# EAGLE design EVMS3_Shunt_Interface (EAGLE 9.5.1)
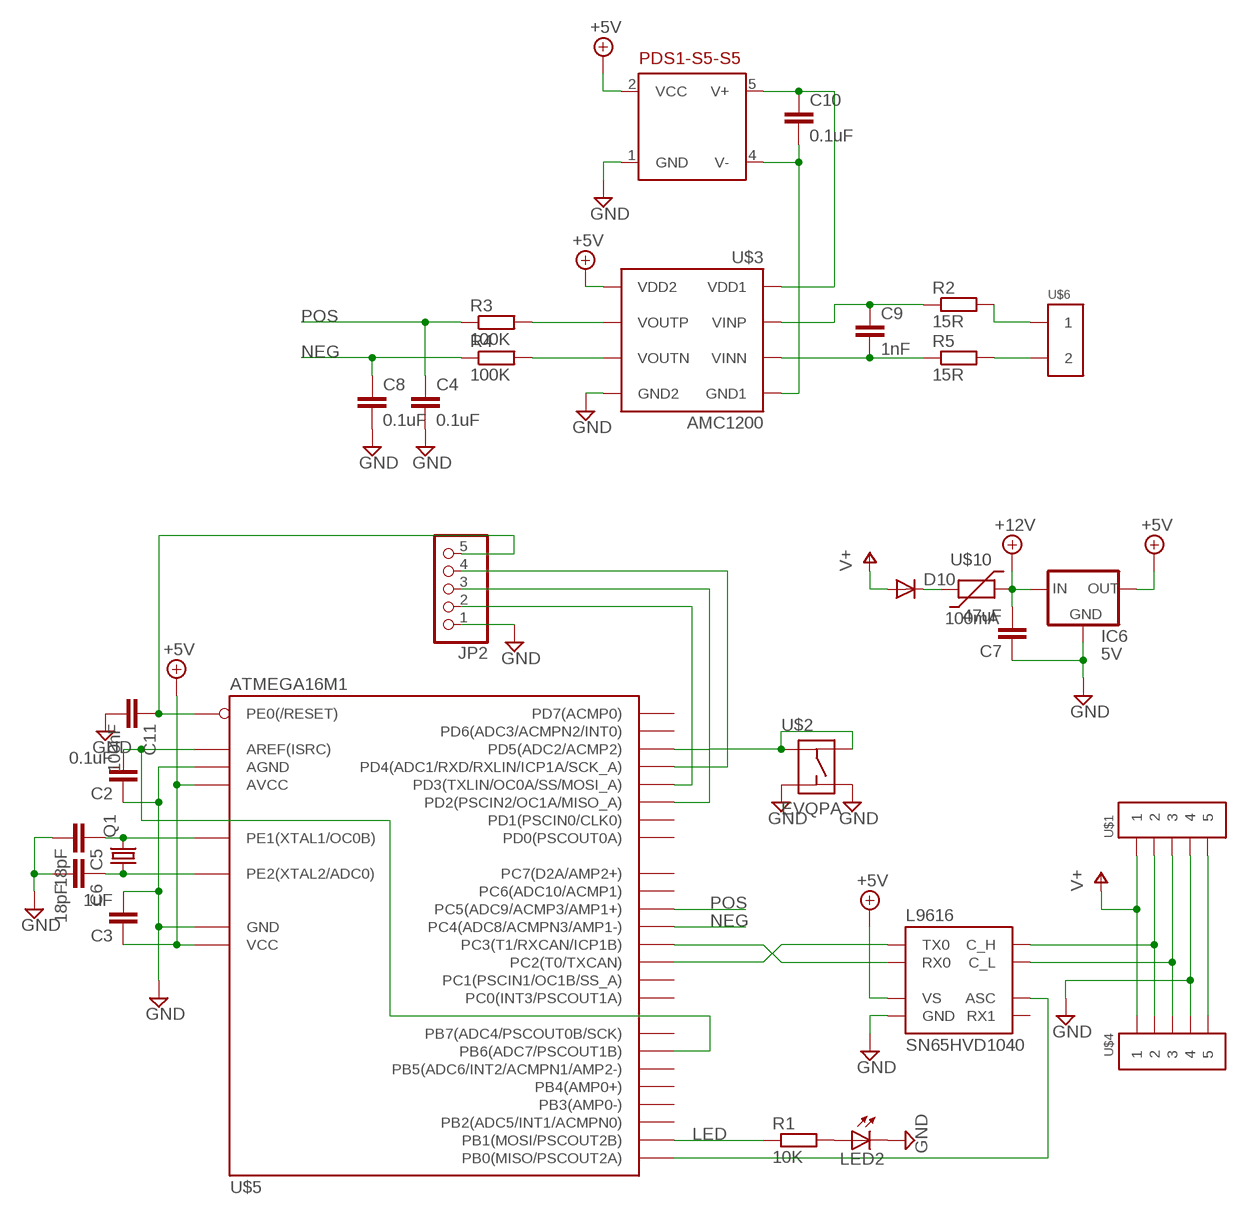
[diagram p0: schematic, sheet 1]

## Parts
C2  0.1uF  C-EUC1206  [C1206]
C3  1uF  C-EUC1206  [C1206]
C4  0.1uF  C-EUC1206  [C1206]
C5  18pF  C-EUC0805  [C0805]
C6  18pF  C-EUC0805  [C0805]
C7  47uF  C-EUC1206  [C1206]
C8  0.1uF  C-EUC1206  [C1206]
C9  1nF  C-EUC1206  [C1206]
C10  0.1uF  C-EUC1206  [C1206]
C11  100nF  C-EUC1206  [C1206]
D10  DIODE-SOD123  [SOD123]
IC6  5V  78LXXSOT89  [SOT89R]
JP2  PINHD-1X5  [1X05]
LED2  LED3MM  [LED3MM]
PDS1-S5-S5  PDS2  [PDS2]
Q1  CRYSTALCTS406  [CTS406]
R1  10K  R-EU_R1206  [R1206]
R2  15R  R-EU_R1206  [R1206]
R3  100K  R-EU_R1206  [R1206]
R4  100K  R-EU_R1206  [R1206]
R5  15R  R-EU_R1206  [R1206]
SN65HVD1040  L9616  [SOIC8]
U$1  MOLEX-39502-1005  [MOLEX-39502-1005]
U$2  EVQPA  [EVQPA]
U$3  AMC1200  [SOIC8W]
U$4  MOLEX-39502-1005  [MOLEX-39502-1005]
U$5  ATMEGA16M1  [TQFP32]
U$6  MOLEX-39502-1002  [MOLEX-39502-1002]
U$10  100mA  1206_POLYSWITCH  [1206]

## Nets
+5V: C3.1 IC6.2(OUT) PDS1-S5-S5.2(VCC) SN65HVD1040.P$3(VS) U$3.8(VDD2) U$5.4(VCC) U$5.19(AVCC)
+12V: C7.2 IC6.1(IN) U$10.P$2
BUTTON: U$2.B U$2.B2 U$5.13(PD5(ADC2/ACMP2))
GND: C2.1 C3.2 C4.2 C5.2 C6.2 C7.1 C8.2 C11.2 IC6.4(GND) JP2.1 LED2.K(C) PDS1-S5-S5.1(GND) SN65HVD1040.P$2(GND) U$1.4 U$2.A U$2.A2 U$3.5(GND2) U$4.4 U$5.5(GND) U$5.20(AGND)
LED: R1.1 U$5.9(PB1(MOSI/PSCOUT2B))
N$1: LED2.A R1.2
N$2: U$1.5 U$4.5
N$3: SN65HVD1040.P$8(ASC) U$5.8(PB0(MISO/PSCOUT2A))
N$4: R4.2 U$3.6(VOUTN)
N$6: C9.2 R5.1 U$3.3(VINN)
N$7: SN65HVD1040.P$7(C_H) U$1.2 U$4.2
N$8: R5.2 U$6.2
N$9: R2.2 U$6.1
N$10: SN65HVD1040.P$6(C_L) U$1.3 U$4.3
N$11: C9.1 R2.1 U$3.2(VINP)
N$12: SN65HVD1040.P$1(TX0) U$5.6(PC2(T0/TXCAN))
N$13: C10.1 PDS1-S5-S5.5(V+) U$3.1(VDD1)
N$14: C10.2 PDS1-S5-S5.4(V-) U$3.4(GND1)
N$15: D10.C U$10.P$1
N$17: SN65HVD1040.P$4(RX0) U$5.7(PC3(T1/RXCAN/ICP1B))
N$18: R3.2 U$3.7(VOUTP)
N$21: C6.1 Q1.1 U$5.11(PE2(XTAL2/ADC0))
N$34: C5.1 Q1.3 U$5.10(PE1(XTAL1/OC0B))
N$42: C2.2 U$5.21(AREF(ISRC)) U$5.27(PB6(ADC7/PSCOUT1B))
N$44: C11.1 JP2.5 U$5.31(PE0(/RESET))
NEG: C8.1 R4.1 U$5.17(PC4(ADC8/ACMPN3/AMP1-))
OUT1: JP2.2 U$5.2(PD3(TXLIN/OC0A/SS/MOSI_A))
OUT2: JP2.3 U$5.1(PD2(PSCIN2/OC1A/MISO_A))
OUT3: JP2.4 U$5.12(PD4(ADC1/RXD/RXLIN/ICP1A/SCK_A))
POS: C4.1 R3.1 U$5.18(PC5(ADC9/ACMP3/AMP1+))
V+: D10.A U$1.1 U$4.1
Unconnected: SN65HVD1040.P$5(RX1) U$5.3(PC1(PSCIN1/OC1B/SS_A)) U$5.14(PD6(ADC3/ACMPN2/INT0)) U$5.15(PD7(ACMP0)) U$5.16(PB2(ADC5/INT1/ACMPN0)) U$5.22(PC6(ADC10/ACMP1)) U$5.23(PB3(AMP0-)) U$5.24(PB4(AMP0+)) U$5.25(PC7(D2A/AMP2+)) U$5.26(PB5(ADC6/INT2/ACMPN1/AMP2-)) U$5.28(PB7(ADC4/PSCOUT0B/SCK)) U$5.29(PD0(PSCOUT0A)) U$5.30(PC0(INT3/PSCOUT1A)) U$5.32(PD1(PSCIN0/CLK0))

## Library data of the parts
C2-C11 = resistor:C-EU: CAPACITOR, European symbol
D10 = diode:DIODE-: DIODE
IC6 = v-reg:78LXX: VOLTAGE REGULATOR
JP2 = pinhead:PINHD-1X5: PIN HEADER
LED2 = led:LED: LED
PDS1-S5-S5 = Ians parts:PDS2
Q1 = crystal:CRYSTAL: CRYSTAL
R1-R5 = resistor:R-EU_: RESISTOR, European symbol
SN65HVD1040 = Ians parts:L9616
U$1 U$4 = Ians parts:MOLEX-39502-1005
U$2 = Ians parts:EVQPA
U$3 = Ians parts:AMC1200
U$5 = Ians parts:ATMEGA16M1
U$6 = Ians parts:MOLEX-39502-1002
U$10 = Ians parts:1206_POLYSWITCH

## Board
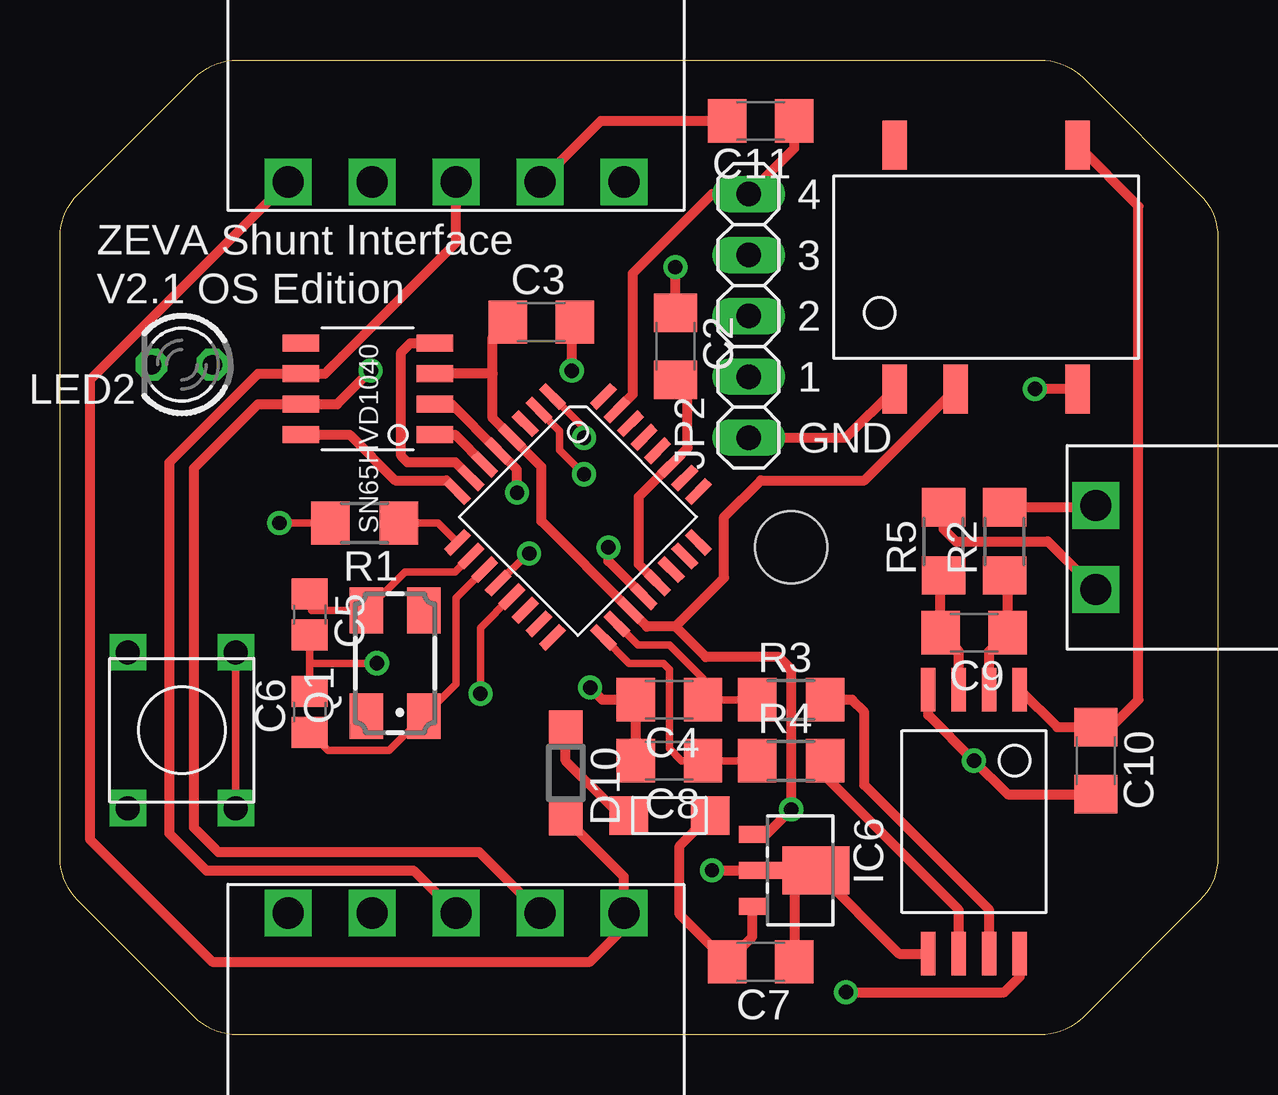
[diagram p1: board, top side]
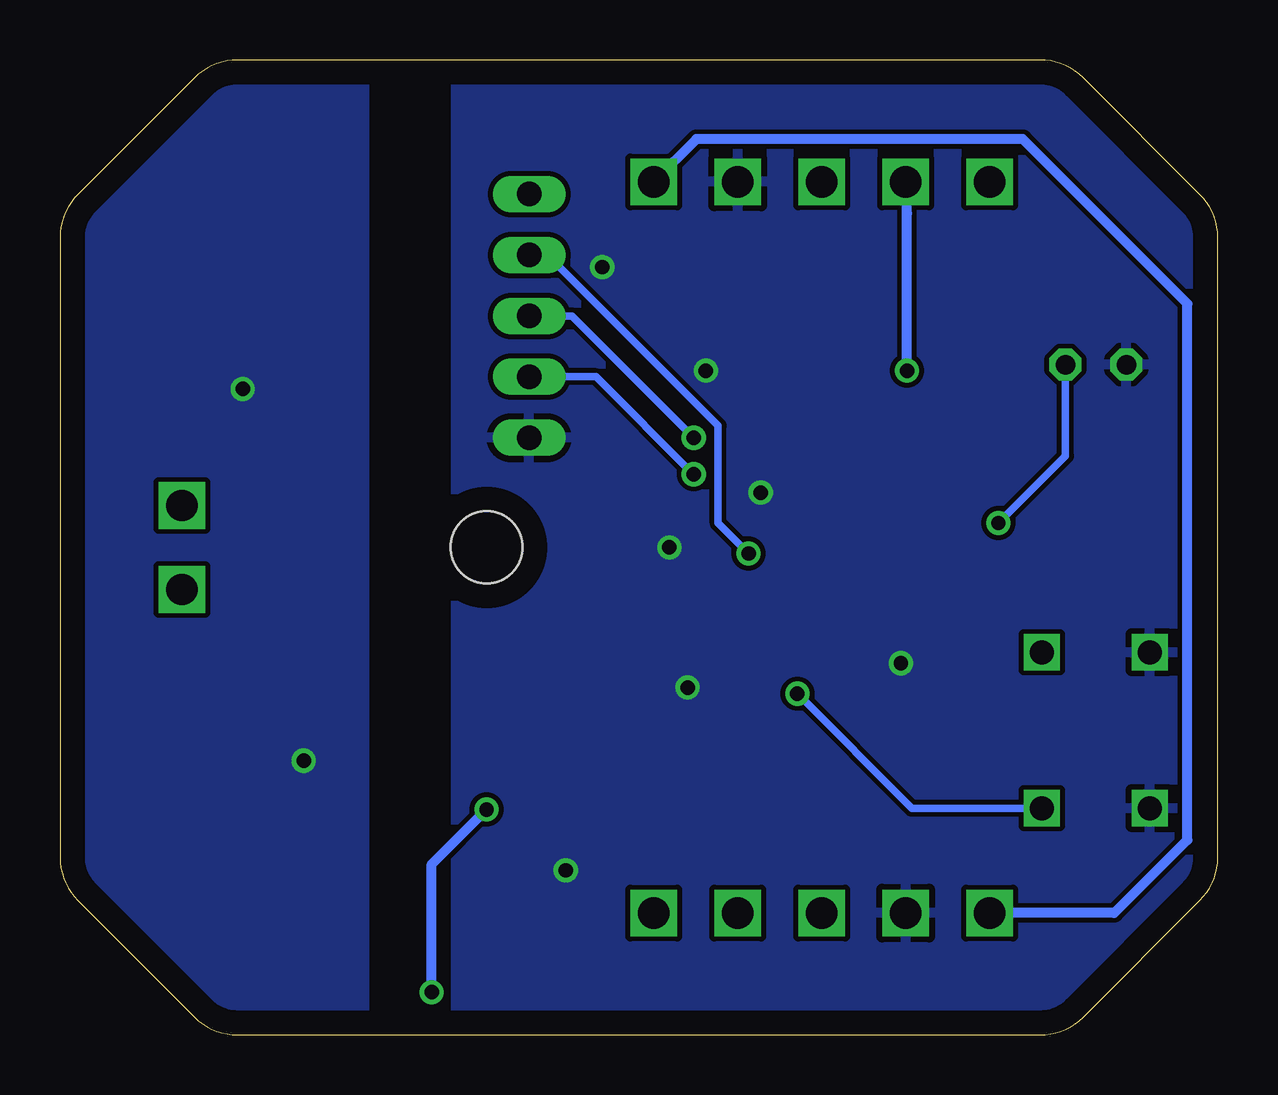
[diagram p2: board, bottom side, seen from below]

Size 48.26 x 40.64 mm. Coordinates in mm from the lower left corner, seen from the top.
Outline: 42.65,0.74 arc-45 40.86,0 7.4,0 arc-45 5.61,0.74 0.74,5.61 arc-45 0,7.4 0,33.24 arc-45 0.74,35.03 5.61,39.9 arc-45 7.4,40.64 40.86,40.64 arc-45 42.65,39.9 47.52,35.03 arc-45 48.26,33.24 48.26,7.4 arc-45 47.52,5.61 42.65,0.74
Copper layers (1*16): Top 0.035mm / dielectric 1.5mm / Bottom 0.035mm
Design rules "default *": minimum track width 10mil, minimum drill 20mil, track to track 8mil, track to pad 8mil, pad to pad 8mil, via to via 8mil, smd to smd 8mil, copper to edge 40mil, drill to drill 8mil, minimum pad ring 10mil, minimum via ring 8mil, stop-mask expansion 4mil, vias tented up to drill 0mil, thermal gap 10mil
Holes 3 mm at 30.48,20.32

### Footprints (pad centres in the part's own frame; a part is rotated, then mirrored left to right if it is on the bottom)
C1206 = smd 1.6 x 1.8: 1 -1.4,0; 2 1.4,0
C0805 = smd 1.3 x 1.5: 1 -0.85,0; 2 0.85,0
SOD123 = smd 1.4 x 1.4: A 1.9,0; C -1.9,0
SOT89R = smd 0.7 x 1.1: 1 1.5,-1.75; 2 -1.5,-1.75 | smd 0.7 x 1.8: 3 0,-1.4 | smd 2 x 2.8: 4 0,0.9
1X05 = drill 1.016 long: 1 -5.08,0; 2 -2.54,0; 3 0,0; 4 2.54,0; 5 5.08,0
LED3MM = drill 0.813 octagon: A -1.27,0; K 1.27,0
PDS2 = smd 1.016 x 2.032: 1 -3.81,-5.08; 2 -1.27,-5.08; 4 3.81,-5.08; 5 3.81,5.08; 8 -3.81,5.08
CTS406 = smd 1.9 x 1.4: 1 -2.2,-1.2; 2 2.2,-1.2; 3 2.2,1.2; 4 -2.2,1.2
R1206 = smd 1.6 x 1.803: 1 -1.422,0; 2 1.422,0
SOIC8 = smd 1.524 x 0.711: P$1 -2.794,1.905; P$2 -2.794,0.635; P$3 -2.794,-0.635; P$4 -2.794,-1.905; P$5 2.794,-1.905; P$6 2.794,-0.635; P$7 2.794,0.635; P$8 2.794,1.905
MOLEX-39502-1005 = drill 1.3 square: 1 -7,0; 2 -3.5,0; 3 0,0; 4 3.5,0; 5 7,0
EVQPA = drill 1 square: A -2.25,3.25; A2 -2.25,-3.25; B 2.25,3.25; B2 2.25,-3.25
SOIC8W = smd 1.8 x 0.6: 1 -5.5,1.905; 2 -5.5,0.635; 3 -5.5,-0.635; 4 -5.5,-1.905; 5 5.5,-1.905; 6 5.5,-0.635; 7 5.5,0.635; 8 5.5,1.905
TQFP32 = smd 1.2 x 0.4: 1 -4.3,2.8; 2 -4.3,2; 3 -4.3,1.2; 4 -4.3,0.4; 5 -4.3,-0.4; 6 -4.3,-1.2; 7 -4.3,-2; 8 -4.3,-2.8; 17 4.3,-2.8; 18 4.3,-2; 19 4.3,-1.2; 20 4.3,-0.4; 21 4.3,0.4; 22 4.3,1.2; 23 4.3,2; 24 4.3,2.8 | smd 0.4 x 1.2: 9 -2.8,-4.3; 10 -2,-4.3; 11 -1.2,-4.3; 12 -0.4,-4.3; 13 0.4,-4.3; 14 1.2,-4.3; 15 2,-4.3; 16 2.8,-4.3; 25 2.8,4.3; 26 2,4.3; 27 1.2,4.3; 28 0.4,4.3; 29 -0.4,4.3; 30 -1.2,4.3; 31 -2,4.3; 32 -2.8,4.3
MOLEX-39502-1002 = drill 1.3 square: 1 -1.75,0; 2 1.75,0
1206 = smd 1.6 x 1.6: P$1 -1.7,0; P$2 1.7,0

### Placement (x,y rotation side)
C2  25.65,28.7 270 top
C3  20.07,29.72 0 top
C4  25.4,13.97 180 top
C5  10.41,17.53 270 top
C6  10.41,13.46 90 top
C7  29.21,3.05 180 top
C8  25.4,11.43 180 top
C9  38.1,16.76 180 top
C10  43.18,11.43 270 top
C11  29.21,38.1 180 top
D10  21.08,10.92 270 top
IC6  30.61,6.86 270 top
JP2  28.7,29.97 90 top
LED2  5.08,27.94 180 top
PDS1-S5-S5  38.61,32 0 top
Q1  13.97,15.49 90 top
R1  12.7,21.34 180 top
R2  39.37,20.57 90 top
R3  30.48,13.97 0 top
R4  30.48,11.43 0 top
R5  36.83,20.57 90 top
SN65HVD1040  12.83,26.92 180 top
U$1  16.51,35.56 0 top
U$2  5.08,12.7 0 top
U$3  38.1,8.89 270 top
U$4  16.51,5.08 180 top
U$5  21.59,21.59 315 top
U$6  43.18,20.32 270 top
U$10  25.4,9.14 0 top

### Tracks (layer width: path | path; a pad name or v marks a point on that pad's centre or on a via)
+5V  (via drill 0.6)
  Top 0.406: IC6.2 29.44,8.36 v30.48,9.4 30.48,15.24 29.97,15.75 26.92,15.75 25.65,17.02 | U$3.8 40.01,2.41 39.37,1.78 v32.77,1.78 | PDS1-S5-S5.2 33.53,23.11 29.21,23.11 27.69,21.59 27.69,19.05 25.65,17.02 | 18.03,27.56 18.03,29.09 C3.1 | 18.03,27.56 SN65HVD1040.P$3 | 18.03,27.56 18.03,25.71 U$5.4 20.07,23.68 20.07,21.42 U$5.19 24.46,17.02 25.65,17.02
  Bottom 0.406: v30.48,9.4 32.77,7.11 v32.77,1.78
+12V
  Top 0.406: 28.76,5.46 IC6.1 28.86,4.09 C7.2 25.83,5.03 25.83,7.87 U$10.P$2
BUTTON  (via drill 0.6)
  Top 0.305: U$2.B2 U$2.B | U$5.13 17.53,16.96 v17.53,14.22
  Bottom 0.305: U$2.B2 12.75,9.45 v17.53,14.22
GND  (via drill 0.6)
  Top 0.305: C6.2 10.41,15.49 | 10.41,15.49 C5.2 | 10.41,15.49 v13.21,15.49
  Top 0.406: C8.2 C4.2 22.61,13.97 v22.1,14.48 | U$5.20 22.86,19.75 v22.86,20.32 | v19.05,22.61 19.05,23.56 U$5.5 16.32,26.29 SN65HVD1040.P$2 | U$3.5 34.98,3.39 IC6.4 30.61,6.86 | JP2.1 32.77,24.89 PDS1-S5-S5.1 | 30.61,6.86 C7.1 | v27.18,6.86 30.61,6.86 | C11.2 22.55,38.1 U$1.4 | C2.1 v25.65,32 | C3.2 21.34,29.59 v21.34,27.69
  pour Bottom: -1.27,-0.64 31.75,-0.64 31.75,41.27 -1.27,41.27
LED
  Top 0.305: R1.1 15.76,21.34 U$5.9
N$1  (via drill 0.6)
  Top 0.305: v9.14,21.34 R1.2
  Bottom 0.305: LED2.A 6.35,24.13 v9.14,21.34
N$2
  Bottom 0.406: U$4.5 4.32,5.08 1.27,8.13 1.27,30.48 8.13,37.34 21.73,37.34 U$1.5
N$3
  Top 0.406: U$5.8 16.11,23.11 13.97,23.11 12.06,25.02 SN65HVD1040.P$8
N$4
  Top 0.406: U$3.6 37.47,5.21 31.9,10.77 R4.2
N$6
  Top 0.406: U$3.3 37.47,16 C9.2 36.7,19.02 R5.1
N$7  (via drill 0.6)
  Top 0.406: v12.95,27.69 11.56,26.29 SN65HVD1040.P$7 8.26,26.29 5.59,23.62 5.59,8.64 6.6,7.62 17.47,7.62 U$4.2
  Bottom 0.406: U$1.2 12.95,34.23 v12.95,27.69
N$8
  Top 0.406: R5.2 36.83,21.08 37.34,20.57 41.18,20.57 U$6.2
N$9
  Top 0.406: R2.2 43.25,22 U$6.1
N$10
  Top 0.406: U$1.3 16.51,33.02 11.05,27.56 SN65HVD1040.P$6 8.26,27.56 4.57,23.88 4.57,8.38 6.1,6.86 14.73,6.86 U$4.3
N$11
  Top 0.406: U$3.2 38.73,16 C9.1 39.5,19.02 R2.1
N$12
  Top 0.406: SN65HVD1040.P$1 16.46,25.02 U$5.6
N$13
  Top 0.406: U$3.1 41.56,12.83 C10.1 43.82,12.83 44.96,13.97 44.96,34.54 PDS1-S5-S5.5
N$14  (via drill 0.6)
  Top 0.406: PDS1-S5-S5.4 v40.64,26.92 | C10.2 39.5,10.03 v38.1,11.43 36.2,13.34 U$3.4
  pour Bottom: 35.56,41.91 49.53,41.91 49.53,-1.27 35.56,-1.27
N$15
  Top 0.406: D10.C 21.08,11.43 23.11,9.4 23.45,9.4 U$10.P$1
N$17
  Top 0.406: U$5.7 16.48,23.88 14.48,23.88 14.22,24.13 14.22,28.45 14.61,28.83 SN65HVD1040.P$4
N$18
  Top 0.406: U$3.7 38.73,5.21 33.53,10.41 33.53,13.46 33.02,13.97 R3.2
N$21
  Top 0.305: U$5.11 16.51,18.21 16.51,14.63 Q1.1 13.73,11.85 11.18,11.85 C6.1
N$34
  Top 0.305: U$5.10 16.48,19.3 14.38,19.3 Q1.3 10.49,17.69 C5.1
N$42
  Top 0.406: U$5.21 24.13,19.62 24.13,22.43 U$5.27 26.16,24.46 26.16,26.92 25.78,27.3 C2.2
N$44
  Top 0.406: C11.1 30.61,36.96 JP2.5 27.18,35.05 23.88,31.75 23.88,26.7 U$5.31
NEG
  Top 0.305: R4.1 C8.1 25.91,11.43 25.4,11.94 25.4,15.24 25.15,15.49 23.73,15.49 U$5.17
OUT1  (via drill 0.6)
  Top 0.305: U$5.2 20.83,25.18 20.83,24.38 v21.84,23.37
  Bottom 0.305: JP2.2 25.91,27.43 v21.84,23.37
OUT2  (via drill 0.6)
  Top 0.305: U$5.1 21.84,25.3 v21.84,24.89
  Bottom 0.305: JP2.3 26.92,29.97 v21.84,24.89
OUT3  (via drill 0.6)
  Top 0.305: v19.56,20.07 19.5,20.07 U$5.12
  Bottom 0.305: v19.56,20.07 20.83,21.34 20.83,25.4 27.94,32.51 JP2.4
POS
  Top 0.305: R3.1 C4.1 26.8,14.86 25.4,16.26 24.1,16.26 U$5.18
V+
  Top 0.406: U$1.1 1.27,27.32 1.27,8.13 6.35,3.05 22.1,3.05 23.51,4.46 U$4.1 23.51,6.59 D10.A

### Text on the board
tPlace: 4 | ZEVA Shunt Interface | 3 | V2.1 OS Edition | 2 | 1 | GND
